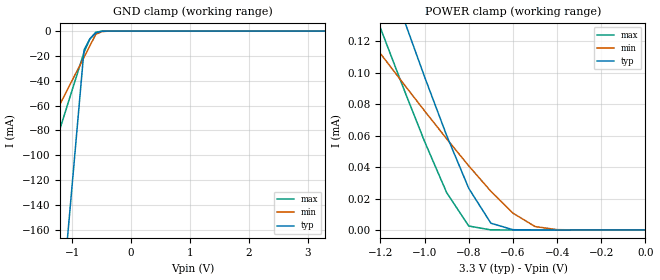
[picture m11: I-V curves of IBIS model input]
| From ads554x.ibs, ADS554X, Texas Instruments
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|   Model input
[Model]   input
Model_type   Terminator
C_comp   3.433pF   3.0333pF   3.8pF
[Temperature Range]   27.00   125.00   -40.00
[Voltage Range]   3.30V   3.00V   3.60V
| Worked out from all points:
|   GND clamp passes 1 mA (typ) near -0.56 V on its own axis
|   POWER clamp passes 1 mA (typ) near -3.17 V on its own axis
[GND_clamp]
| voltage   I(typ)   I(min)   I(max)
-3.3V     -1.364A    -252.3mA   -394.4mA
-2.3V     -824.7mA   -159.9mA   -243.5mA
-1.8V     -554.9mA   -113.6mA   -168mA
-1.7V     -500.9mA   -104.4mA   -152.9mA
-1.1V     -177.1mA   -48.87mA   -62.4mA
-1V       -123.2mA   -39.62mA   -47.31mA
-800mV    -15.24mA   -21.12mA   -17.12mA
-700mV    -6.255mA   -11.87mA   -6.303mA
-600mV    -1.547mA   -2.623mA   -1.01mA
-500mV    -175uA     -522.3uA   -58.5uA
-400mV    -11.65uA   -71.5uA    -1.597uA
3.3V      46.1pA     17.2nA     2.955pA
[POWER_clamp]
| voltage   I(typ)   I(min)   I(max)
-3.3V     1.053mA    512.9uA    940.5uA
-1.3V     216.6uA    130.7uA    165.8uA
-1.2V     176.2uA    112.2uA    128.5uA
-1.1V     136.3uA    93.84uA    91.72uA
-1V       97.34uA    75.72uA    56.19uA
-900mV    60uA       57.96uA    23.67uA
-800mV    26.42uA    40.76uA    2.513uA
-700mV    4.307uA    24.61uA    30.63nA
-600mV    164.1nA    10.7uA     225.4pA
-500mV    3.786nA    2.183uA    7.067pA
-400mV    134.1pA    195.3nA    5.208pA
0V        46.1pA     5.236nA    3.907pA
[Rpower]   11000   12096   9526
[Rgnd]   9167   12096   6804
| End [Model] input
